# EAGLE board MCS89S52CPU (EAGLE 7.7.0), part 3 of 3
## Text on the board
tPlace: EXT-PORT | GND | C024H | C028H | C02CH | C030H | C034H | C038H | C03CH | ADR0 | ADR1 | RD | WR | ADR8 | ADR9 | ADR10 | ADR11 | ADR12 | ADR13 | ADR14 | ADR15 | GND | DB0 | DB1 | DB2 | DB3 | DB4 | DB5 | DB6 | DB7 | ALE-OUT | INT1 | INT0 | DMA-A | RESET | CLK | CI | CO | LPO | GND | VCC | J.L. | RESET | O-M-S-U | ADDRESS-LATCH | MCS52-BASIC MCU | V1.1 - V1.31 | IO-DECODER | V1.2 | NVRAM | RAM | FLASH | CLOCK | MCU | DECODER | PIO | - | PSU | PWM-OUT | + | PA0 | PB4 | PB3 | VCC | PA1 | PA2 | PA3 | PA4 | PA5 | PA6 | PA7 | PC0 | PC1 | PC2 | PC3 | PC4 | PC5 | PC6 | PC7 | PB7 | PB6 | PB5 | PB2 | PB1 | PB0 | RES-IN | GND | VCC | PWM | P10 | P11 | T0/SCL | T1/SDA | PROG-EN | RESET | GND | LPO | CO | CI | GND | USER-PORT
tNames: * | EA | FS | FD | FP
